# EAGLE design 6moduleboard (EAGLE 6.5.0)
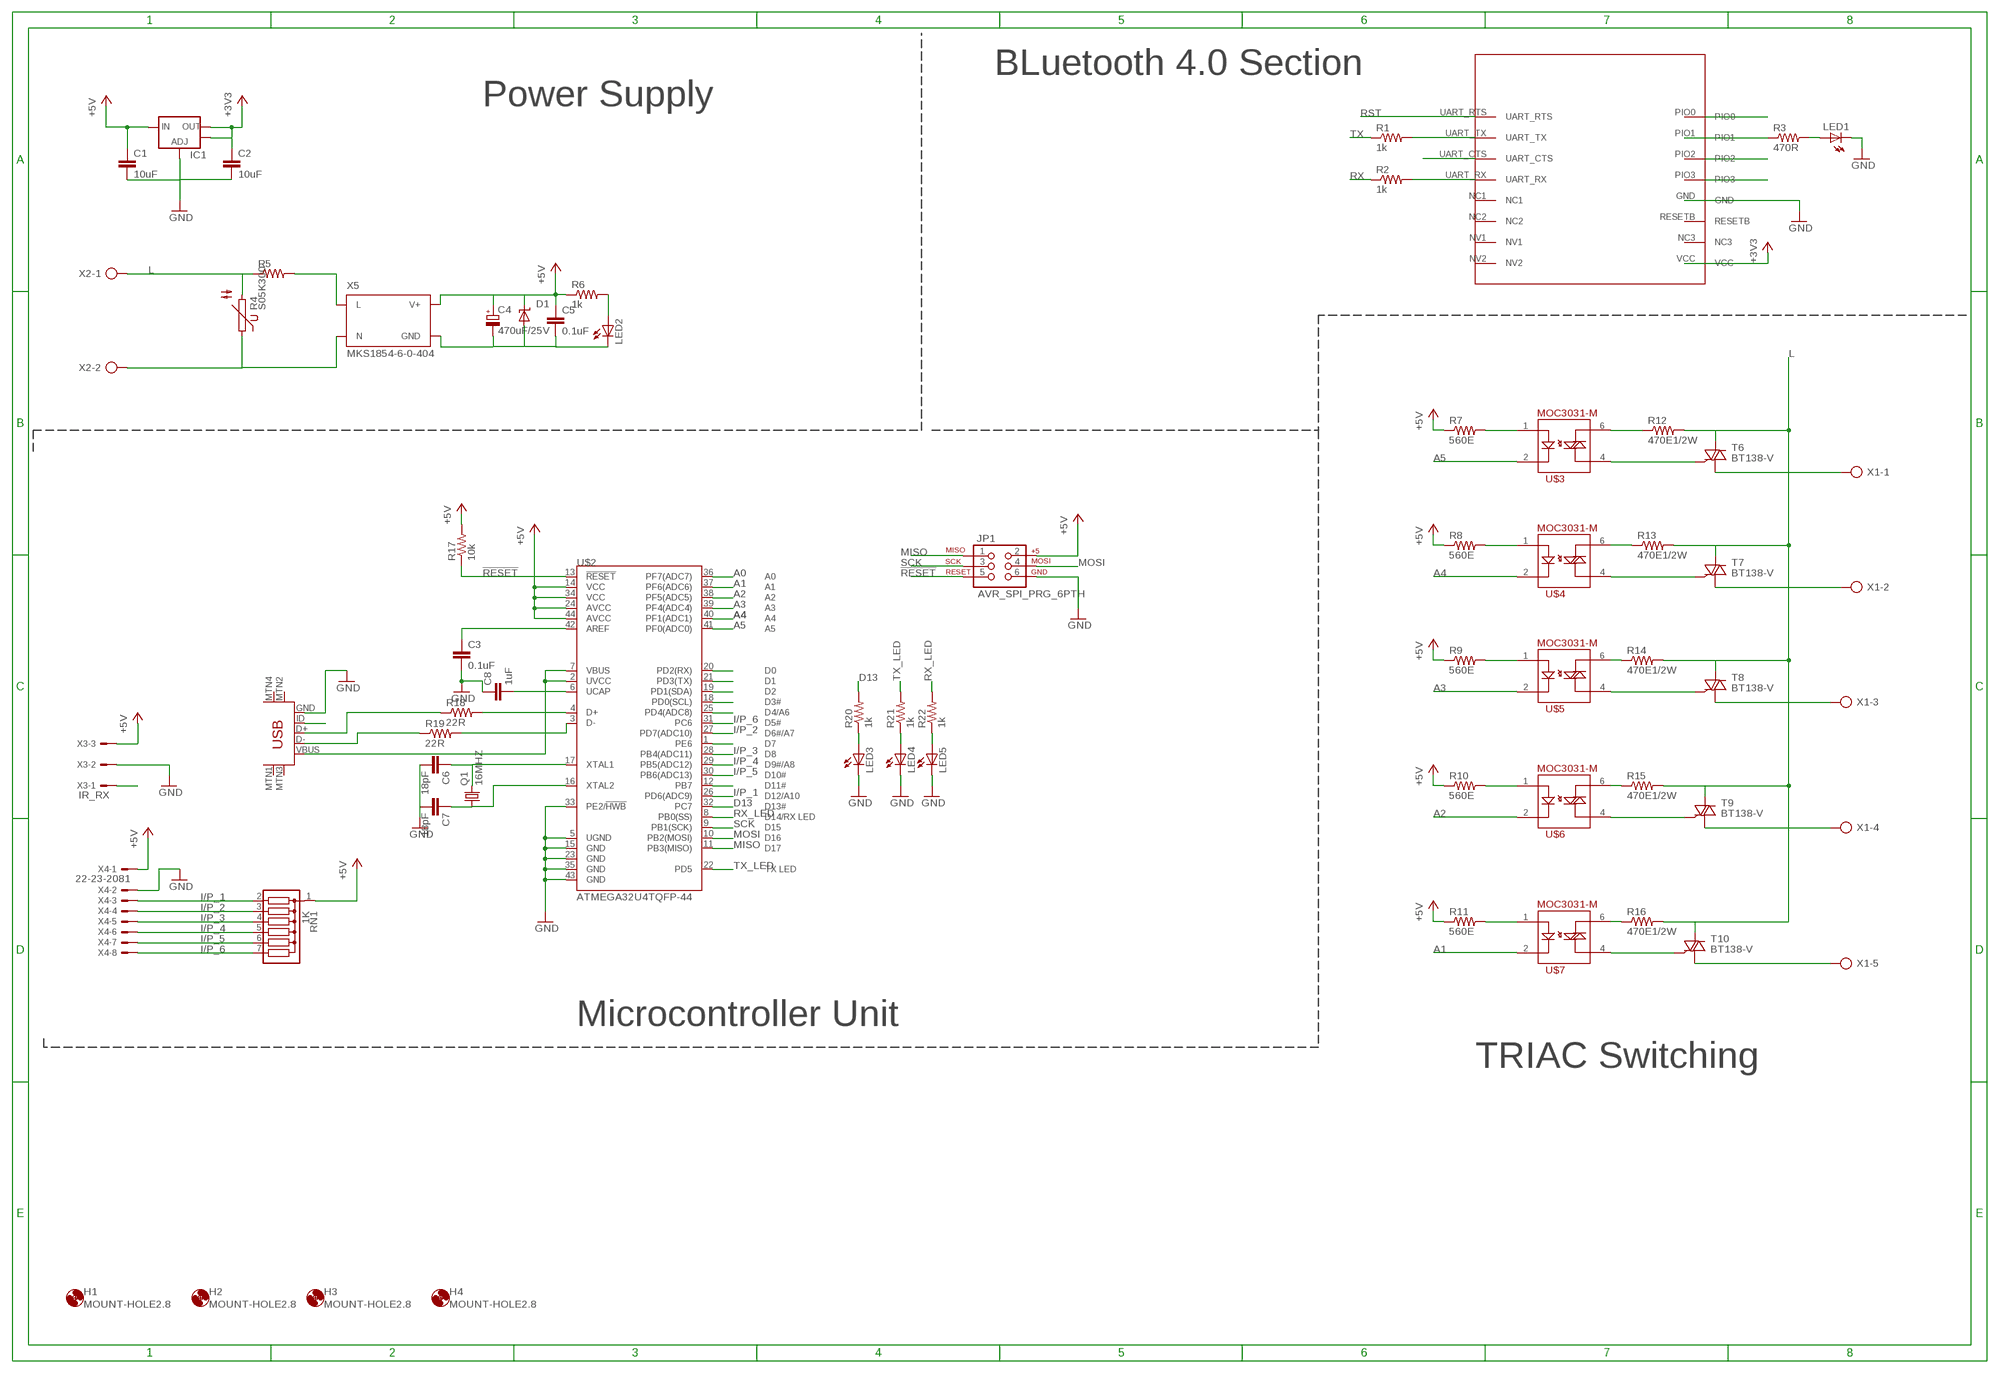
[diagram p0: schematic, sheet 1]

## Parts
C1  10uF  10UF-6.3V-20%(1206)  [1206]
C2  10uF  10UF-6.3V-20%(1206)  [1206]
C3  0.1uF  CAP1206  [1206]
C4  470uF/25V  CPOL-EUE5-8.5  [E5-8,5]
C5  0.1uF  1.0UF50V10%(1206)  [1206]
C6  18pF  CAP1206  [1206]
C7  18pF  CAP1206  [1206]
C8  1uF  CAP1206  [1206]
D1  SUPPRESSOR-SMBJ  [SMBJ]
H1  MOUNT-HOLE2.8  [2,8]
H2  MOUNT-HOLE2.8  [2,8]
H3  MOUNT-HOLE2.8  [2,8]
H4  MOUNT-HOLE2.8  [2,8]
IC1  V_REG_LM1117SOT223  [SOT223]
JP1  AVR_SPI_PRG_6PTH  [2X3]
LED1  LEDSMT1206  [1206]
LED2  LEDSMT1206  [1206]
LED3  LEDSMT1206  [1206]
LED4  LEDSMT1206  [1206]
LED5  LEDSMT1206  [1206]
Q1  16MHZ  CRYSTALHC49UP  [HC49UP]
R1  1k  RESISTOR1206  [1206]
R2  1k  RESISTOR1206  [1206]
R3  470R  RESISTOR1206  [1206]
R4  S05K300  [S05K300]
R5  R-US_0207/10  [0207/10]
R6  1k  RESISTOR1206  [1206]
R7  560E  RESISTOR1206  [1206]
R8  560E  RESISTOR1206  [1206]
R9  560E  RESISTOR1206  [1206]
R10  560E  RESISTOR1206  [1206]
R11  560E  RESISTOR1206  [1206]
R12  470E1/2W  R-US_0411/3V  [0411V]
R13  470E1/2W  R-US_0411/3V  [0411V]
R14  470E1/2W  R-US_0411/3V  [0411V]
R15  470E1/2W  R-US_0411/3V  [0411V]
R16  470E1/2W  R-US_0411/3V  [0411V]
R17  10k  RESISTOR1206  [1206]
R18  22R  RESISTOR1206  [1206]
R19  22R  RESISTOR1206  [1206]
R20  1k  RESISTOR1206  [1206]
R21  1k  RESISTOR1206  [1206]
R22  1k  RESISTOR1206  [1206]
RN1  1K  G06R  [SIL7]
T6  BT138-V  [TO220BV]
T7  BT138-V  [TO220BV]
T8  BT138-V  [TO220BV]
T9  BT138-V  [TO220BV]
T10  BT138-V  [TO220BV]
U$1  HM-11  [HM-11]
U$2  ATMEGA32U4TQFP-44  [TQFP44]
U$3  MOC3083  MOC3031-M  [DIL06]
U$4  MOC3083  MOC3031-M  [DIL06]
U$5  MOC3083  MOC3031-M  [DIL06]
U$6  MOC3083  MOC3031-M  [DIL06]
U$7  MOC3083  MOC3031-M  [DIL06]
U$8  USB-MINIB-5PIN  [USB-MINIB]
X1  AK300/5  [AK300/5]
X2  AK300/2  [AK300/2]
X3  IR_RX  22-23-2031  [22-23-2031]
X4  22-23-2081  [22-23-2081]
X5  MKS1854-6-0-404  [MKS1854-6-0-404]

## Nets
!RESET: JP1.5 R17.1 U$2.13(!RESET)
+3V3: C2.1 IC1.2(OUT) IC1.4(OUT) U$1.VCC
+5V: C1.1 C4.+ C5.1 D1.C IC1.3(IN) JP1.2 R6.1 R7.1 R8.1 R9.1 R10.1 R11.1 R17.2 RN1.1 U$2.14(VCC) U$2.24(AVCC) U$2.34(VCC) U$2.44(AVCC) X3.3 X4.1 X5.3(V+)
A0: U$2.36(PF7(ADC7))
A1: U$2.37(PF6(ADC6)) U$7.2
A2: U$2.38(PF5(ADC5)) U$6.2
A3: U$2.39(PF4(ADC4)) U$5.2
A4: U$2.40(PF1(ADC1)) U$4.2
A5: U$2.41(PF0(ADC0)) U$3.2
D13: R20.2 U$2.32(PC7)
GND: C1.2 C2.2 C3.2 C6.2 C7.2 C8.1 IC1.1(ADJ) JP1.6 LED1.C LED3.C LED4.C LED5.C U$1.GND U$2.5(UGND) U$2.15(GND) U$2.23(GND) U$2.33(PE2/!HWB) U$2.35(GND) U$2.43(GND) U$8.GND X3.2 X4.2
I/P_1: RN1.2 U$2.26(PD6(ADC9)) X4.3
I/P_2: RN1.3 U$2.27(PD7(ADC10)) X4.4
I/P_3: RN1.4 U$2.28(PB4(ADC11)) X4.5
I/P_4: RN1.5 U$2.29(PB5(ADC12)) X4.6
I/P_5: RN1.6 U$2.30(PB6(ADC13)) X4.7
I/P_6: RN1.7 U$2.31(PC6) X4.8
L: R4.2 R5.1 R12.2 R13.2 R14.2 R15.2 R16.2 T6.T2(A2) T7.T2(A2) T8.T2(A2) T9.T2(A2) T10.T2(A2) X2.1
MISO: JP1.1 U$2.11(PB3(MISO))
MOSI: JP1.4 U$2.10(PB2(MOSI))
N$1: R3.1 U$1.PIO1
N$2: LED1.A R3.2
N$3: R5.2 X5.1(L)
N$4: R4.1 X2.2 X5.2(N)
N$5: R1.2 U$1.UART_TX
N$6: U$1.UART_CTS
N$7: R2.2 U$1.UART_RX
N$12: T6.T1(A1) X1.1
N$13: T7.T1(A1) X1.2
N$14: R7.2 U$3.1
N$15: C4.- C5.2 D1.A LED2.C X5.4(GND)
N$16: R12.1 U$3.6
N$17: R8.2 U$4.1
N$18: LED2.A R6.2
N$19: R9.2 U$5.1
N$20: R10.2 U$6.1
N$21: R11.2 U$7.1
N$28: X3.1
N$29: LED4.A R21.1
N$30: LED5.A R22.1
N$31: U$2.20(PD2(RX))
N$32: R13.1 U$4.6
N$33: R14.1 U$5.6
N$34: R15.1 U$6.6
N$35: R16.1 U$7.6
N$36: U$2.21(PD3(TX))
N$37: T6.G U$3.4
N$38: U$2.25(PD4(ADC8))
N$39: T7.G U$4.4
N$41: T8.G U$5.4
N$42: C8.2 U$2.6(UCAP)
N$43: T9.G U$6.4
N$44: C3.1 U$2.42(AREF)
N$45: T10.G U$7.4
N$46: T10.T1(A1) X1.5
N$47: T8.T1(A1) X1.3
N$48: T9.T1(A1) X1.4
N$49: U$2.19(PD1(SDA))
N$50: R18.2 U$2.4(D+)
N$51: R19.2 U$2.3(D-)
N$52: R18.1 U$8.D+
N$53: R19.1 U$8.D-
N$54: C6.1 Q1.2 U$2.17(XTAL1)
N$55: C7.1 Q1.1 U$2.16(XTAL2)
N$56: U$2.18(PD0(SCL))
N$68: U$2.12(PB7)
N$72: U$2.1(PE6)
N$80: LED3.A R20.1
N$81: U$8.ID
N$84: U$2.2(UVCC) U$2.7(VBUS) U$8.VBUS
RST: U$1.UART_RTS
RX: R2.1
RX_LED: R22.2 U$2.8(PB0(SS))
SCK: JP1.3 U$2.9(PB1(SCK))
TX: R1.1
TX_LED: R21.2 U$2.22(PD5)
Unconnected: U$1.NC1 U$1.NC2 U$1.NC3 U$1.NV1 U$1.NV2 U$1.PIO0 U$1.PIO2 U$1.PIO3 U$1.RESETB U$8.MTN1(MTN2) U$8.MTN2(MTN3) U$8.MTN3(MTN1) U$8.MTN4

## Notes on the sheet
- BLuetooth 4.0 Section
- Power Supply
- Microcontroller Unit
- TRIAC Switching

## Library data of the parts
C1 C2 = SparkFun-Capacitors:10UF-6.3V-20%(1206): CAP-10057; PROD_ID: CAP-10057
C3 C6-C8 = SparkFun-Passives:CAP: Capacitor
C4 = rcl:CPOL-EU: POLARIZED CAPACITOR, European symbol
C5 = SparkFun-Capacitors:1.0UF50V10%(1206): CAP-09822; PROD_ID: CAP-09822; VALUE: 1.0uF
D1 = diode:SUPPRESSOR-: Suppressor diode
H1-H4 = holes:MOUNT-HOLE: MOUNTING HOLE with drill center marker
IC1 = SparkFun-PowerIC:V_REG_LM1117: Voltage Regulator LM1117 Standard adjustable voltage regulator but in SMD form. Spark Fun Electronics SKU : COM-00595; PROD_ID: VREG-08170
JP1 = SparkFun-Connectors:AVR_SPI_PRG_6: AVR ISP 6 Pin This is the reduced ISP connector for AVR programming. Common on Arduino. This footprint will take up less PCB space and can be used with a 10-pin to 6-pin adapter such as SKU: BOB-08508 **Special note about "TEST_POINT" package. The stop mask is on the top side, so if you want your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
LED1-LED5 = led:LED: LED
Q1 = crystal:CRYSTAL: CRYSTAL; OC_FARNELL: unknown; OC_NEWARK: unknown
R1-R3 R6 R17-R22 = SparkFun-Passives:RESISTOR: Resistor
R4 = varistor:S05K300: VARISTOR
R5 R12-R16 = rcl:R-US_: RESISTOR, American symbol
R7-R11 = SparkFun-Resistors:RESISTOR: Resistor
RN1 = resistor-sil:G06R: SIL RESISTOR; OC_FARNELL: unknown; OC_NEWARK: unknown
T6-T10 = triac:BT138: TRIAC Source: http://www.semiconductors.philips.com BT138_SERIES_2.pdf
U$1 = HM-11:HM-11
U$2 = SparkFun-DigitalIC:ATMEGA32U4: Atmel 44-pin 8-bit Microcontroller with 32KBytes of ISP Flash and USB Controller
U$3-U$7 = SparkFun-DiscreteSemi:MOC3031-M: Opto-isolated TRIAC
U$8 = SparkFun-Connectors:USB-MINIB: Mini-USB "B" connector with 5th pin broken out. Created new symbol breaking out 5th "ID" pin in mini/micro USB connector spec. See: http://en.wikipedia.org/wiki/Mini_usb#Cables. Uses same footprint as 4-pin symbol. Also added pins to connect to mounting / shield pads if required (probably not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
X1 = con-ptr500:AK300/5: CONNECTOR; OC_FARNELL: unknown; OC_NEWARK: unknown
X2 = con-ptr500:AK300/2: CONNECTOR; OC_FARNELL: unknown; OC_NEWARK: unknown
X3 = con-molex:22-23-2031: .100" (2.54mm) Center Header - 3 Pin; MF: MOLEX; MPN: 22-23-2031; OC_FARNELL: 1462950; OC_NEWARK: 30C0862
X4 = con-molex:22-23-2081: .100" (2.54mm) Center Header - 8 Pin; MF: MOLEX; MPN: 22-23-2081; OC_FARNELL: 1756826; OC_NEWARK: 01C7592
X5 = Morsun-con-stocko:MKS1854-6-0-404: Serie MKS 1850 Lötstifte In-line, Raster 2.5 mm, Stiftwannen, stehend, mit Rastlasche Source: http://www.stocko.de/de/index.php?seite=ka_rfk2_mks1850.html&rubrik=Katalog+-+RFK+2 rfk_1850.pdf; OC_FARNELL: 1141862; OC_NEWARK: unknown

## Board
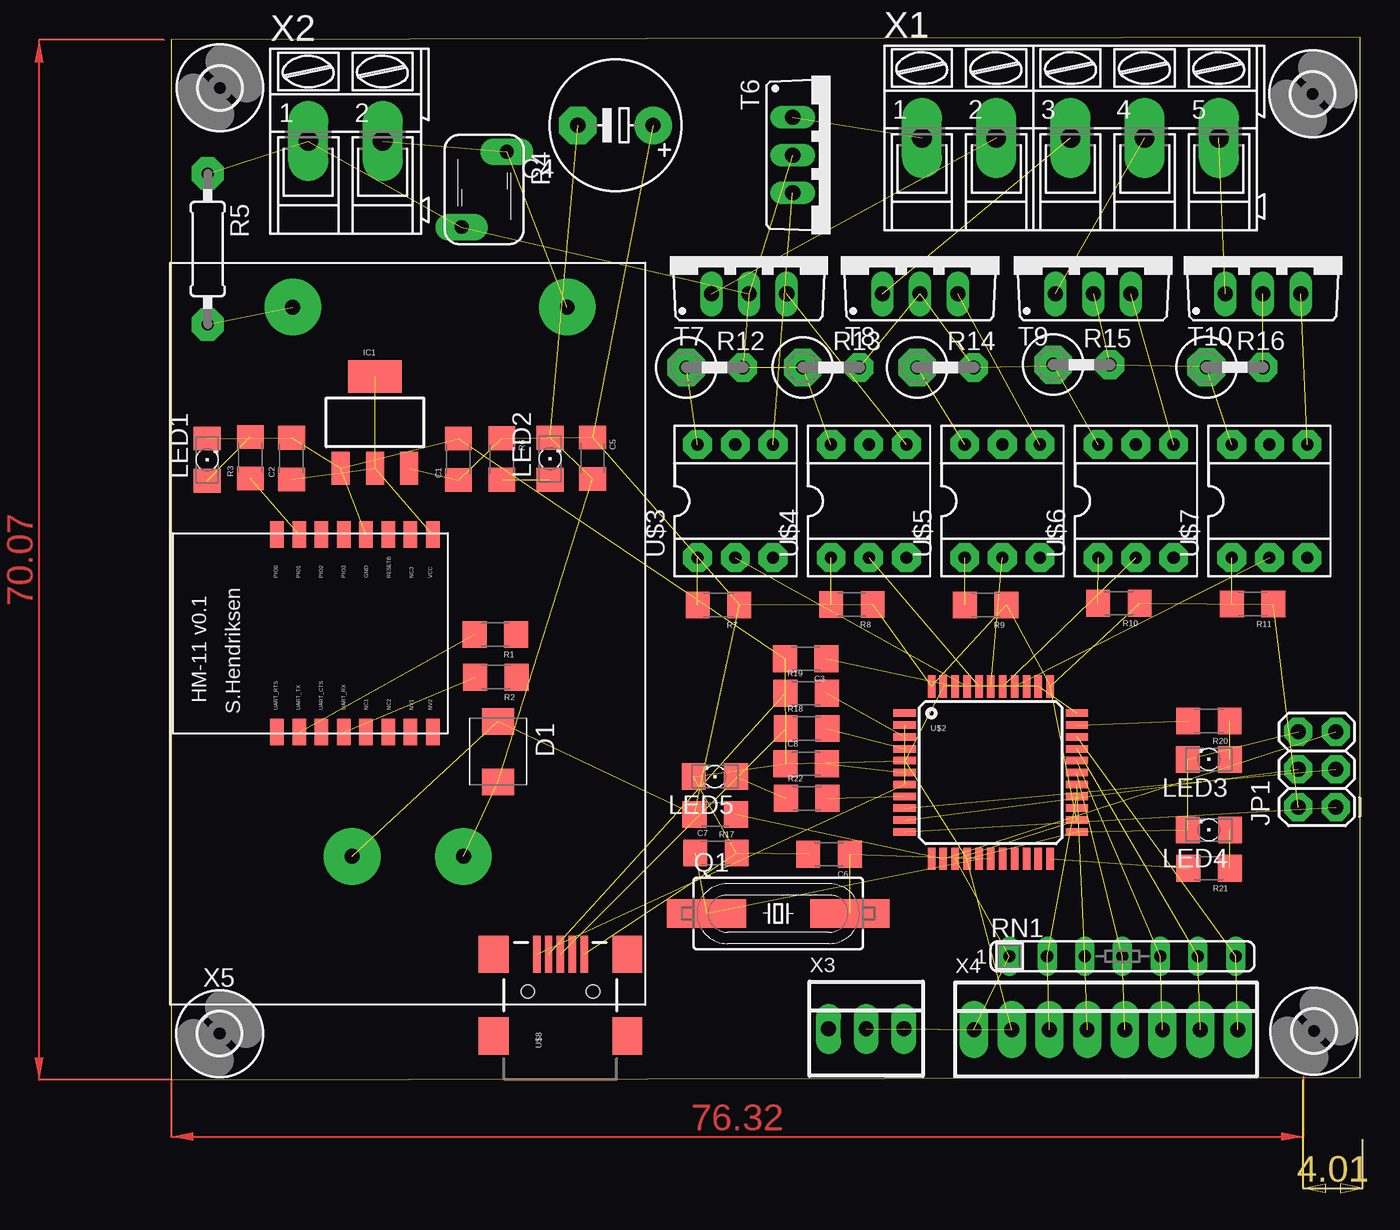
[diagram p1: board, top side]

Size 80.29 x 77.84 mm. Coordinates in mm from the lower left corner, seen from the top.
Outline: 0,7.58 80.16,7.77 80.16,77.84 0,77.64 0,7.58
Copper layers (1*16): Top 0.035mm / dielectric 1.5mm / Bottom 0.035mm
Design rules "default": minimum track width 10mil, minimum drill 24mil, track to track 8mil, track to pad 8mil, pad to pad 8mil, via to via 8mil, smd to smd 8mil, copper to edge 40mil, drill to drill 8mil, minimum pad ring 10mil, minimum via ring 8mil, stop-mask expansion 4mil, vias tented up to drill 0mil, thermal gap 10mil

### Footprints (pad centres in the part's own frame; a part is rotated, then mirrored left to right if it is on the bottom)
1206 = smd 1.6 x 1.8: 1 -1.4,0; 2 1.4,0
E5-8,5 = drill 1.016 pad 2.54: + -2.54,0 | drill 1.016 pad 2.54 octagon: - 2.54,0
SMBJ = smd 1.78 x 2.16: A 2.04,0; C -2.03,0
2,8 = hole 2.8: 0,0
SOT223 = smd 1.219 x 2.235: 1 -2.311,-3.099; 2 0,-3.099; 3 2.311,-3.099 | smd 3.6 x 2.2: 4 0,3.099
2X3 = drill 1.016 pad 1.88 octagon: 1 0,0; 2 0,2.54; 3 2.54,0; 4 2.54,2.54; 5 5.08,0; 6 5.08,2.54
1206' = smd 1.6 x 1.803: A -1.422,0; C 1.422,0
HC49UP = smd 5.334 x 1.93: 1 -4.826,0; 2 4.826,0
S05K300 = drill 0.914 pad 1.778 long: 1 -1.524,-2.54; 2 1.524,2.54
0207/10 = drill 0.8 pad 2.184 octagon: 1 -5.08,0; 2 5.08,0
0411V = drill 0.914 pad 2.54 octagon: 1 -2.54,0 | drill 0.914 pad 1.93 octagon: 2 1.27,0
SIL7 = drill 0.813 long: 1 -7.62,0; 2 -5.08,0; 3 -2.54,0; 4 0,0; 5 2.54,0; 6 5.08,0; 7 7.62,0
TO220BV = drill 1.016 long: G 2.54,-2.54; T1 -2.54,-2.54; T2 0,-2.54
HM-11 = smd 1.778 x 0.914: GND 7.508,-0.6; NC1 -5.808,-0.6; NC2 -5.808,-2.1; NC3 7.508,-3.6; NV1 -5.808,-3.6; NV2 -5.808,-5.1; PIO0 7.508,5.4; PIO1 7.508,3.9; PIO2 7.508,2.4; PIO3 7.508,0.9; RESETB 7.508,-2.1; UART_CTS -5.808,2.4; UART_RTS -5.808,5.4; UART_RX -5.808,0.9; UART_TX -5.808,3.9; VCC 7.508,-5.1
TQFP44 = smd 1.5 x 0.5: 1 -5.8,4; 2 -5.8,3.2; 3 -5.8,2.4; 4 -5.8,1.6; 5 -5.8,0.8; 6 -5.8,0; 7 -5.8,-0.8; 8 -5.8,-1.6; 9 -5.8,-2.4; 10 -5.8,-3.2; 11 -5.8,-4; 23 5.8,-4; 24 5.8,-3.2; 25 5.8,-2.4; 26 5.8,-1.6; 27 5.8,-0.8; 28 5.8,0; 29 5.8,0.8; 30 5.8,1.6; 31 5.8,2.4; 32 5.8,3.2; 33 5.8,4 | smd 0.5 x 1.5: 12 -4,-5.8; 13 -3.2,-5.8; 14 -2.4,-5.8; 15 -1.6,-5.8; 16 -0.8,-5.8; 17 0,-5.8; 18 0.8,-5.8; 19 1.6,-5.8; 20 2.4,-5.8; 21 3.2,-5.8; 22 4,-5.8; 34 4,5.8; 35 3.2,5.8; 36 2.4,5.8; 37 1.6,5.8; 38 0.8,5.8; 39 0,5.8; 40 -0.8,5.8; 41 -1.6,5.8; 42 -2.4,5.8; 43 -3.2,5.8; 44 -4,5.8
DIL06 = drill 0.813 pad 1.93 octagon: 1 -3.51,-3.81; 2 -0.97,-3.81; 3 1.57,-3.81; 4 1.57,3.81; 5 -0.97,3.81; 6 -3.51,3.81
USB-MINIB = smd 2.5 x 0.5: D+ 2.5,0; D- 2.5,0.8; GND 2.5,-1.6; ID 2.5,-0.8; VBUS 2.5,1.6 | smd 2.5 x 2: MTN1 -3,4.5; MTN2 2.5,4.5; MTN3 -3,-4.5; MTN4 2.5,-4.5 | hole 0.9: 0,2.2; 0,-2.2
AK300/5 = drill 1.321 pad 2.7 long: 1 -10.008,0; 2 -5.004,0; 3 0,0; 4 5.004,0; 5 10.008,0
AK300/2 = drill 1.321 pad 2.7 long: 1 -2.515,0; 2 2.489,0
22-23-2031 = drill 1 pad 1.676 long: 1 -2.54,0; 2 0,0; 3 2.54,0
22-23-2081 = drill 1 pad 1.93 long: 1 -8.89,0; 2 -6.35,0; 3 -3.81,0; 4 -1.27,0; 5 1.27,0; 6 3.81,0; 7 6.35,0; 8 8.89,0
MKS1854-6-0-404 = drill 1 pad 3.81: 1 8.25,47; 2 26.75,47; 3 12.25,10; 4 19.75,10

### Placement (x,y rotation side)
C1  19.37,49.39 90 top
C2  8.13,49.44 90 top
C3  42.78,35.96 180 top
C4  29.96,71.89 180 top
C5  28.42,49.47 270 top
C6  44.35,22.79 180 top
C7  36.73,22.87 0 top
C8  42.81,28.89 0 top
D1  22.04,29.71 270 top
H1  3.3,74.42 0 top
H2  76.95,74.01 0 top
H3  3.28,10.71 0 top
H4  77.03,10.88 0 top
IC1  13.75,51.88 0 top
JP1  78.51,25.96 90 top
LED1  [1206']  2.44,49.37 90 top
LED2  [1206']  25.55,49.43 90 top
LED3  [1206']  69.94,29.17 180 top
LED4  [1206']  69.95,24.42 180 top
LED5  [1206']  36.65,28.02 180 top
Q1  40.93,18.8 0 top
R1  21.86,37.59 180 top
R2  21.9,34.72 180 top
R3  5.35,49.5 90 top
R4  21.11,67.57 180 top
R5  2.48,63.56 270 top
R6  22.3,49.42 270 top
R7  36.9,39.58 180 top
R8  45.89,39.61 180 top
R9  54.9,39.58 180 top
R10  63.88,39.7 180 top
R11  72.9,39.64 180 top
R12  37.27,55.58 0 top
R13  45.12,55.58 0 top
R14  52.83,55.58 0 top
R15  62,55.77 0 top
R16  72.32,55.59 0 top
R17  36.68,25.47 180 top
R18  42.84,31.25 0 top
R19  42.81,33.63 0 top
R20  69.95,31.77 180 top
R21  69.96,21.84 180 top
R22  42.85,26.55 0 top
RN1  64.13,15.91 0 top
T6  44.44,69.89 270 top
T7  38.96,63.08 0 top
T8  50.48,63.08 0 top
T9  62.15,63.08 0 top
T10  73.59,63.08 0 top
U$1  12.54,36.82 90 top
U$2  55.25,28.29 0 top
U$3  39,46.58 0 top
U$4  48,46.58 0 top
U$5  57,46.58 0 top
U$6  66,46.58 0 top
U$7  75,46.58 0 top
U$8  26.25,13.54 90 top
X1  60.62,71.05 0 top
X2  11.78,70.82 0 top
X3  46.85,11.02 0 top
X4  63.01,10.97 0 top
X5  -0.04,12.65 0 top

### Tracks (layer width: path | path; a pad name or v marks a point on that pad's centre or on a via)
!RESET  (2 unrouted)
+3V3  (3 unrouted)
+5V  (20 unrouted)
  Top 0.203: IC1.3 15.58,47.99
A1  (1 unrouted)
A2  (1 unrouted)
A3  (1 unrouted)
A4  (1 unrouted)
A5  (1 unrouted)
D13  (1 unrouted)
GND  (21 unrouted)
I/P_1  (2 unrouted)
I/P_2  (2 unrouted)
I/P_3  (2 unrouted)
I/P_4  (2 unrouted)
I/P_5  (2 unrouted)
I/P_6  (2 unrouted)
L  (12 unrouted)
MISO  (1 unrouted)
MOSI  (1 unrouted)
N$1  (1 unrouted)
N$2  (1 unrouted)
N$3  (1 unrouted)
N$4  (2 unrouted)
N$5  (1 unrouted)
N$7  (1 unrouted)
N$12  (1 unrouted)
N$13  (1 unrouted)
N$14  (1 unrouted)
N$15  (4 unrouted)
N$16  (1 unrouted)
N$17  (1 unrouted)
N$18  (1 unrouted)
N$19  (1 unrouted)
N$20  (1 unrouted)
N$21  (1 unrouted)
N$29  (1 unrouted)
N$30  (1 unrouted)
N$32  (1 unrouted)
N$33  (1 unrouted)
N$34  (1 unrouted)
N$35  (1 unrouted)
N$37  (1 unrouted)
N$39  (1 unrouted)
N$41  (1 unrouted)
N$42  (1 unrouted)
N$43  (1 unrouted)
N$44  (1 unrouted)
N$45  (1 unrouted)
N$46  (1 unrouted)
N$47  (1 unrouted)
N$48  (1 unrouted)
N$50  (1 unrouted)
N$51  (1 unrouted)
N$52  (1 unrouted)
N$53  (1 unrouted)
N$54  (2 unrouted)
N$55  (2 unrouted)
N$80  (1 unrouted)
N$84  (2 unrouted)
RX_LED  (1 unrouted)
SCK  (1 unrouted)
TX_LED  (1 unrouted)
(copper drawn outside any net)
  shapes: Top area x2

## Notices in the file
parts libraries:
SparkFun-PowerIC: Licensing: Creative Commons ShareAlike 4.0 International - https://creativecommons.org/licenses/by-sa/4.0
